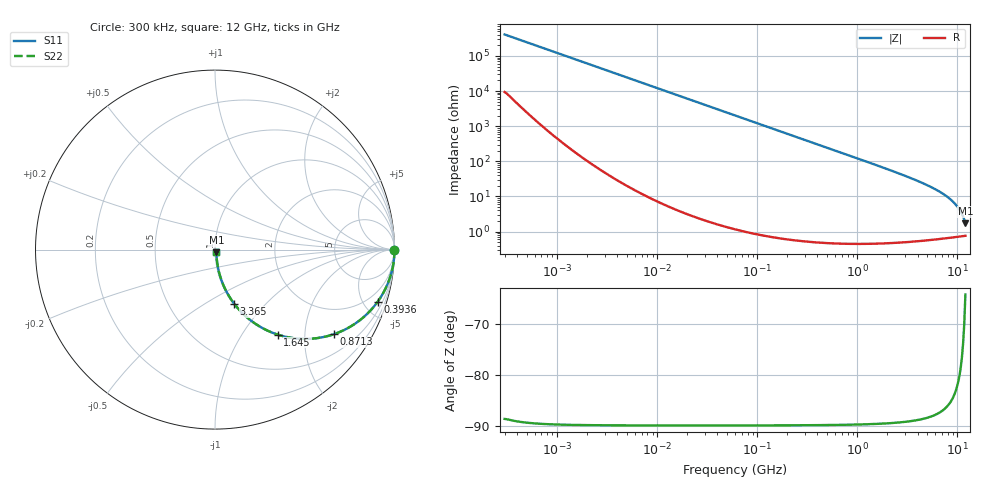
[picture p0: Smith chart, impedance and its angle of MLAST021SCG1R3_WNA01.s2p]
! MLAST021SCG1R3_WNA01  S-PARAMETER MODEL  ( General Type )
! Model Generated by TAIYO YUDEN Corporation (http://www.ty-top.com)
! Version 1.0
! TAIYO YUDEN Control No. 220901
! Copyright(c) 2022 TAIYO YUDEN CO.,LTD. All Rights Reserved.
! Product Description (link to TY-COMPAS)
! https://ds.yuden.co.jp/TYCOMPAS/or/detail?pn=MLAST021SCG1R3BWNA01&u=M
! Products Name : Multilayer Ceramic Capacitors
! Characteristics :
!  Capacitance : 1.3 pF , Rated Voltage : 25V , TCC : CG / C0G
!  Case Size : 0.25 x 0.125 / 0.0098 x 0.0049 [mm/inch] , Thickness : 0.125 / 0.0049 [mm/inch]
!  (Conditions: Temperature = 25 degC , DC Bias Current/Voltage = 0A / 0V)
! External Node Assignments :
!  1  o---| |---o  2
! GND o---------o GND
! Frequency Range : 0.3MHz  -  12000MHz  [ 401 STEP ]
# MHz S RI R 50
! Freq[MHz].  S11 Real  S11 Imag  S21 Real  S21 Imag  S12 Real  S12 Imag  S22 Real  S22 Imag
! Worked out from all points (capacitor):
!   401 points, 300 kHz to 12 GHz, reference 50 ohm
!   read as one part in series: C = 1.3 pF near 316.3 kHz
!   lowest |Z| = 1.74 ohm at 12 GHz (marker M1)
!   S11 on the Smith chart (normalised r, x): 300 kHz: open; 393.6 MHz: 1.01, -6.22; 871.3 MHz: 1.01, -2.80; 1.645 GHz: 1.01, -1.46; 3.365 GHz: 1.01, -0.68; 12 GHz: 1.02, -0.03
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0.3  1 -0.000245  5.69e-06 0.000245  5.69e-06 0.000245  1 -0.000245
1.769972  1 -0.00145  4.83e-06 0.00145  4.83e-06 0.00145  1 -0.00145
10.44266  0.9999 -0.00853  7.77e-05 0.00853  7.77e-05 0.00853  0.9999 -0.00853
60  0.9976 -0.0489  0.00242 0.0489  0.00242 0.0489  0.9976 -0.0489
159.8975  0.9831 -0.1284  0.0169 0.1284  0.0169 0.1284  0.9831 -0.1284
250.8588  0.9595 -0.1966  0.0405 0.1966  0.0405 0.1966  0.9595 -0.1966
353.9943  0.9224 -0.2668  0.0776 0.2668  0.0776 0.2668  0.9224 -0.2668
393.5654  0.9058 -0.2913  0.0942 0.2913  0.0942 0.2913  0.9058 -0.2913
585.5907  0.8127 -0.3891  0.1873 0.3891  0.1873 0.3891  0.8127 -0.3891
871.3074  0.6613 -0.4717  0.3387 0.4717  0.3387 0.4717  0.6613 -0.4717
1197.383  0.5068 -0.4978  0.4932 0.4978  0.4932 0.4978  0.5068 -0.4978
1645.489  0.3499 -0.4738  0.6501 0.4738  0.6501 0.4738  0.3499 -0.4738
2088.533  0.2478 -0.4276  0.7522 0.4276  0.7522 0.4276  0.2478 -0.4276
3364.605  0.1071 -0.3018  0.8929 0.3018  0.8929 0.3018  0.1071 -0.3018
5565.855  0.0366 -0.1723  0.9634 0.1723  0.9634 0.1723  0.0366 -0.1723
6879.757  0.0221 -0.1248  0.9779 0.1248  0.9779 0.1248  0.0221 -0.1248
8064.993  0.0151 -0.0918  0.9849 0.0918  0.9849 0.0918  0.0151 -0.0918
8966.534  0.0118 -0.0707  0.9882 0.0707  0.9882 0.0707  0.0118 -0.0707
9968.853  0.00958 -0.0503  0.9904 0.0503  0.9904 0.0503  0.00958 -0.0503
10793.46  0.00849 -0.0352  0.9915 0.0352  0.9915 0.0352  0.00849 -0.0352
11686.27  0.00788 -0.0204  0.9921 0.0204  0.9921 0.0204  0.00788 -0.0204
12000  0.00778 -0.0155  0.9922 0.0155  0.9922 0.0155  0.00778 -0.0155
